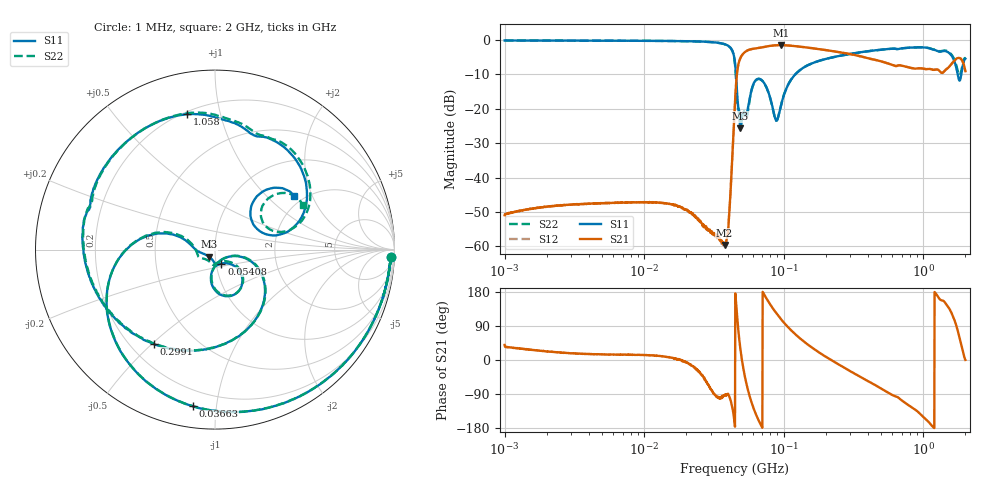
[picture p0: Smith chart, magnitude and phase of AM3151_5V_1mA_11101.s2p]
! Date/Time: Fri Jun 26 11:04:49 2020
! Network Analyzer:  Rev:
! Sweep from 1000000.0 to 2000000000.0, 1601 Points ! Power Supply: 0 V, 0 A
# HZ S DB R 50
!freq MagS11 AngS11 MagS21 AngS21 MagS12 AngS12 MagS22 AngS22
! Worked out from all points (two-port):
!   1601 points, 1 MHz to 2 GHz, reference 50 ohm
!   highest |S21| = -1.51 dB at 95.64 MHz (marker M1); lowest = -59.6 dB at 37.69 MHz (marker M2)
!   |S21| within 3 dB of the highest: 50.05 MHz to 333.1 MHz (283.1 MHz wide, 148 % of centre)
!   lowest |S11| = -25.7 dB at 48.95 MHz (marker M3), VSWR 1.11, Z = 46.7 - j3.76 ohm
!   |S11| at or under -10 dB: 45.44 MHz to 121 MHz (75.51 MHz wide, 90.8 % of centre); 1.761 GHz to 1.87 GHz (109 MHz wide, 6 % of centre)
!   |S22| runs from -23.4 to -0.2 dB; largest |S21 - S12| = 0.0093
!   S11 on the Smith chart (normalised r, x): 1 MHz: 19, -41; 36.63 MHz: 0.11, -0.86; 54.08 MHz: 1.06, -0.17; 299.1 MHz: 0.29, -0.51; 1.058 GHz: 0.21, +0.79; 2 GHz: 1.78, +1.50
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1000000  -0.16 -2.3  -50.95 39.9  -50.70 35.3  -0.16 -2.3
3555161  -0.21 -7.5  -47.68 16.7  -47.71 16.1  -0.20 -7.4
1.263916e7  -0.28 -26.1  -47.27 10.8  -47.34 11.2  -0.29 -26.1
2.457866e7  -0.45 -54.4  -52.55 -32.1  -52.31 -30.6  -0.46 -54.4
3.663215e7  -1.09 -98.0  -59.09 -98.0  -59.03 -96.9  -1.11 -98.4
3.76913e7  -1.24 -103.9  -59.62 -91.8  -59.89 -91.7  -1.25 -104.4
4.047516e7  -1.85 -123.6  -51.90 -94.3  -52.07 -95.5  -1.90 -124.4
4.493426e7  -7.43 172.3  -16.49 175.7  -16.49 175.7  -8.07 168.8
4.894563e7  -25.70 -129.3  -5.21 27.4  -5.21 27.3  -22.61 -130.8
5.108369e7  -21.23 -88.2  -4.04 -18.2  -4.04 -18.2  -21.38 -98.4
5.408043e7  -21.34 -65.1  -3.20 -63.6  -3.20 -63.6  -22.72 -66.4
5.890834e7  -14.30 -42.3  -2.65 -113.1  -2.65 -113.2  -14.51 -39.7
6.857994e7  -11.50 -77.2  -2.22 -171.5  -2.21 -171.5  -11.56 -75.9
8.738118e7  -23.15 -70.0  -1.55 126.0  -1.55 126.0  -23.22 -67.5
9.563502e7  -18.93 -18.5  -1.51 107.4  -1.52 107.4  -18.81 -17.1
1.589914e8  -6.82 -61.5  -2.39 33.0  -2.38 32.9  -6.82 -61.3
2.990693e8  -4.05 -123.0  -4.12 -29.5  -4.12 -29.5  -4.07 -123.5
5.652395e8  -2.62 176.3  -6.91 -87.2  -6.88 -87.1  -2.63 174.4
1.058199e9  -2.26 101.8  -8.50 -158.6  -8.46 -158.9  -2.24 99.4
1.525561e9  -3.77 40.8  -7.86 136.9  -7.88 136.1  -3.56 39.7
1.726123e9  -8.32 13.1  -5.44 89.4  -5.49 88.9  -7.58 14.6
2e9  -5.43 34.2  -9.08 0.3  -9.19 -0.6  -5.22 26.9
